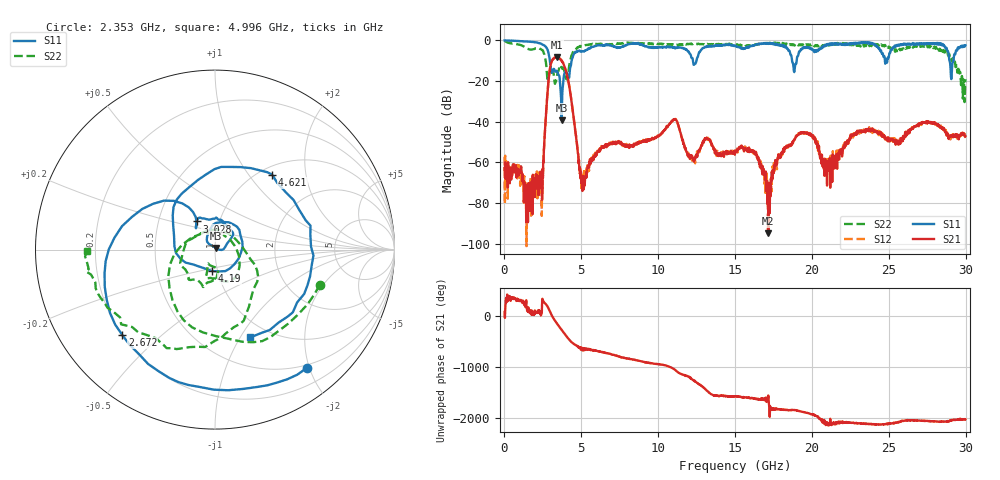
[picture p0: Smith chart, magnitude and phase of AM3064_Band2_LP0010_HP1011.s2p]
# Hz S DB R 50.0
!freq dBS11 angS11 dBS21 angS21 dBS12 angS12 dBS22 angS22
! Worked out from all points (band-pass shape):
!   1600 points, 10 MHz to 29.98 GHz, reference 50 ohm
!   highest |S21| = -8.28 dB at 3.403 GHz (marker M1); lowest = -94.8 dB at 17.16 GHz (marker M2)
!   |S21| within 3 dB of the highest: 3.028 GHz to 3.82 GHz (791.9 MHz wide, 23.1 % of centre)
!   lowest |S11| = -39.3 dB at 3.721 GHz (marker M3), VSWR 1.02, Z = 50.6 + j0.928 ohm
!   |S11| at or under -10 dB: 2.952 GHz to 4.367 GHz (1.415 GHz wide, 38.7 % of centre); 18.71 GHz to 19.01 GHz (297.8 MHz wide, 1.58 % of centre); 28.95 GHz to 29.2 GHz (256.3 MHz wide, 0.881 % of centre)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
!   |S22| runs from -30.4 to -0.2 dB; largest |S21 - S12| = 0.012
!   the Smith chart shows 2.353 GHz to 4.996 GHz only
!   S11 on the Smith chart (normalised r, x): 2.353 GHz: 0.45, -1.97; 2.672 GHz: 0.20, -0.38; 3.028 GHz: 0.78, +0.25; 4.19 GHz: 0.94, -0.23; 4.621 GHz: 1.14, +1.31; 4.996 GHz: 0.81, -1.10
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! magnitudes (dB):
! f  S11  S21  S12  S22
! 10 MHz  0.0  -62.8  -57.2  -0.2
! 2.353 GHz  -1.6  -65.3  -71.1  -4.2
! 2.672 GHz  -3.1  -40.1  -39.9  -9.6
! 3.028 GHz  -14.5  -11.3  -11.3  -15.6
! 3.403 GHz  -15.1  -8.3  -8.5  -18.2
! 3.721 GHz  -39.3  -10.0  -10.0  -13.1
! 4.19 GHz  -18.4  -21.4  -21.6  -13.7
! 4.621 GHz  -5.6  -45.3  -45.2  -4.4
! 4.996 GHz  -5.6  -70.4  -68.8  -2.9
! 5.015 GHz  -5.5  -69.8  -74.1  -2.9
! 10 GHz  -3.5  -47.0  -47.1  -1.8
! 15 GHz  -2.6  -54.8  -55.3  -1.9
! 16.26 GHz  -2.4  -55.7  -55.0  -2.4
! 17.16 GHz  -1.6  -94.8  -76.3  -1.4
! 18.25 GHz  -3.4  -52.9  -53.4  -1.9
! 19.99 GHz  -4.3  -46.5  -46.5  -2.0
! 21.04 GHz  -1.9  -59.2  -58.7  -2.0
! 23.05 GHz  -1.1  -44.4  -45.4  -2.6
! 25 GHz  -8.4  -47.9  -48.8  -3.0
! 28.56 GHz  -2.5  -44.0  -43.6  -4.8
! 29.06 GHz  -19.1  -47.1  -46.1  -8.5
! 29.98 GHz  -2.4  -47.2  -47.0  -19.1
